(* SV subscriber APDU *)
{attribute 'call_after_init'}
{attribute 'analysis' := '-33'}
{attribute 'no_assign'}
{attribute 'no_explicit_call' := 'Direct call not allowed for type FB_SVRXAPDU_IED_MUnn_LLN0_MSVCB02'}
FUNCTION_BLOCK FB_SVRXAPDU_IED_MUnn_LLN0_MSVCB02 EXTENDS FB_GseSvApduClass
VAR_OUTPUT
	RxData: ST_SVAPDU_IED_MUnn_LLN0_MSVCB02; (* Subscribed SV data in TwinCAT PLC host format (little endian) *)
END_VAR
VAR
	Asdu1: ARRAY [0..cOversampleFactor_IED_MUnn_LLN0_MSVCB02_Asdu1-1] OF FB_SVRXASDU_IED_MUnn_LLN0_MSVCB02;
	index: UINT(0..cOversampleFactor_IED_MUnn_LLN0_MSVCB02_Asdu1-1);
END_VAR

{attribute 'call_after_init'}
(* This method adds new oversampling ASDU to the APDU *)
METHOD FINAL AddArrayOfAsduToContainer
VAR
END_VAR
FOR index:=0 TO cOversampleFactor_IED_MUnn_LLN0_MSVCB02_Asdu1-1 BY 1 DO
	Asdu1[index].index:=index;
	Asdu1[index].ipApdu:=THIS^.AddAsduToContainer(ipAsdu:=Asdu1[index]);
END_FOR
END_METHOD

{attribute 'analysis' := '-33'}
(* Converts received SV subscriber data from network (big-endian) to host (little-endian) byte order *)
METHOD FINAL OnSvSubscriberNetToHost
VAR_INPUT
	ipAdapter: I_GseAdapterClass; (* Network adapter interface pointer *)
	ipApdu: I_GseSvApduClass; (* APDU object interface pointer *)
END_VAR
VAR
END_VAR
FOR index:=0 TO cOversampleFactor_IED_MUnn_LLN0_MSVCB02_Asdu1-1 BY 1 DO
	RxData.Asdu1.nSmpCnt[index]:= Asdu1[index].nSmpCnt; (* Get sample counter *)
	RxData.Asdu1.eSmpSynch[index]:= Asdu1[index].eSmpSynch; (* Get synchronization type: 0..2 *)
	RxData.Asdu1.tRefrTm[index]:= Asdu1[index].tRefrTm; (* Get refresh time stamp (optional) *)

	(* Convert received SV data from network byte order to host byte order *)
	NetToHostInt32(in:=Asdu1[index].Values.IED_MUnn_InnATCTR1_AmpSv_instMag_i, out:=RxData.Asdu1.IED_MUnn_InnATCTR1_AmpSv_instMag_i[index]);
	NetToHostQuality(in:=Asdu1[index].Values.IED_MUnn_InnATCTR1_AmpSv_q, out:=RxData.Asdu1.IED_MUnn_InnATCTR1_AmpSv_q[index]);
	NetToHostInt32(in:=Asdu1[index].Values.IED_MUnn_InnBTCTR2_AmpSv_instMag_i, out:=RxData.Asdu1.IED_MUnn_InnBTCTR2_AmpSv_instMag_i[index]);
	NetToHostQuality(in:=Asdu1[index].Values.IED_MUnn_InnBTCTR2_AmpSv_q, out:=RxData.Asdu1.IED_MUnn_InnBTCTR2_AmpSv_q[index]);
	NetToHostInt32(in:=Asdu1[index].Values.IED_MUnn_InnCTCTR3_AmpSv_instMag_i, out:=RxData.Asdu1.IED_MUnn_InnCTCTR3_AmpSv_instMag_i[index]);
	NetToHostQuality(in:=Asdu1[index].Values.IED_MUnn_InnCTCTR3_AmpSv_q, out:=RxData.Asdu1.IED_MUnn_InnCTCTR3_AmpSv_q[index]);
	NetToHostInt32(in:=Asdu1[index].Values.IED_MUnn_InnNTCTR4_AmpSv_instMag_i, out:=RxData.Asdu1.IED_MUnn_InnNTCTR4_AmpSv_instMag_i[index]);
	NetToHostQuality(in:=Asdu1[index].Values.IED_MUnn_InnNTCTR4_AmpSv_q, out:=RxData.Asdu1.IED_MUnn_InnNTCTR4_AmpSv_q[index]);
	NetToHostInt32(in:=Asdu1[index].Values.IED_MUnn_UnnATVTR1_VolSv_instMag_i, out:=RxData.Asdu1.IED_MUnn_UnnATVTR1_VolSv_instMag_i[index]);
	NetToHostQuality(in:=Asdu1[index].Values.IED_MUnn_UnnATVTR1_VolSv_q, out:=RxData.Asdu1.IED_MUnn_UnnATVTR1_VolSv_q[index]);
	NetToHostInt32(in:=Asdu1[index].Values.IED_MUnn_UnnBTVTR2_VolSv_instMag_i, out:=RxData.Asdu1.IED_MUnn_UnnBTVTR2_VolSv_instMag_i[index]);
	NetToHostQuality(in:=Asdu1[index].Values.IED_MUnn_UnnBTVTR2_VolSv_q, out:=RxData.Asdu1.IED_MUnn_UnnBTVTR2_VolSv_q[index]);
	NetToHostInt32(in:=Asdu1[index].Values.IED_MUnn_UnnCTVTR3_VolSv_instMag_i, out:=RxData.Asdu1.IED_MUnn_UnnCTVTR3_VolSv_instMag_i[index]);
	NetToHostQuality(in:=Asdu1[index].Values.IED_MUnn_UnnCTVTR3_VolSv_q, out:=RxData.Asdu1.IED_MUnn_UnnCTVTR3_VolSv_q[index]);
	NetToHostInt32(in:=Asdu1[index].Values.IED_MUnn_UnnNTVTR4_VolSv_instMag_i, out:=RxData.Asdu1.IED_MUnn_UnnNTVTR4_VolSv_instMag_i[index]);
	NetToHostQuality(in:=Asdu1[index].Values.IED_MUnn_UnnNTVTR4_VolSv_q, out:=RxData.Asdu1.IED_MUnn_UnnNTVTR4_VolSv_q[index]);
END_FOR
END_METHOD

END_FUNCTION_BLOCK
